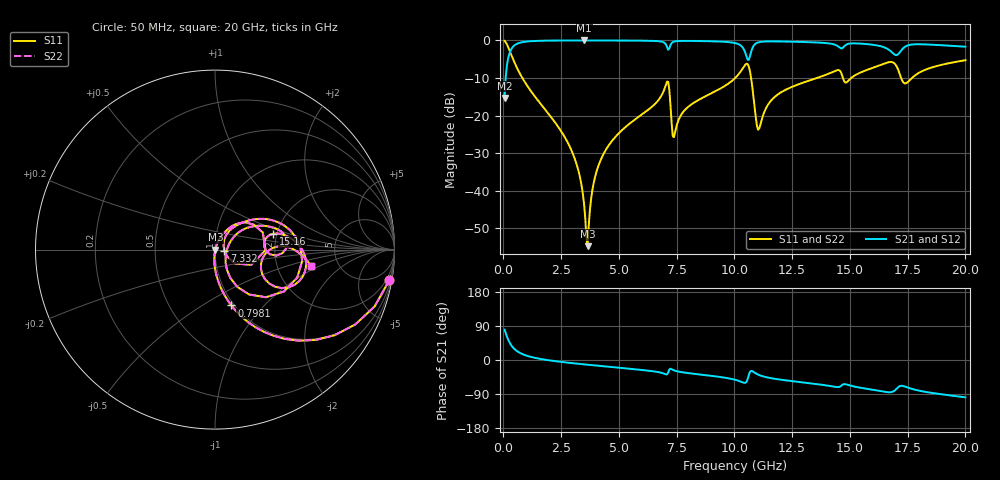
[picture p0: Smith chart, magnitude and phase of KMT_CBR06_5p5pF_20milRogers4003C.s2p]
! Data measured by Modelithics Inc. support@modelithics.com 813-866-6335
! KEMET CBR0603 5.5pF, Pad Width= 0.851mm, Pad Length= 0.64mm, Pad Gap= 0.62mm, 20mil Rogers 4003C substrate Data, January 2022
# hz S ma R 50
! 2 Port Network Data from SP1.SP block
! freq  magS11  angS11  magS21  angS21  magS12  angS12  magS22  angS22
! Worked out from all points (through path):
!   401 points, 50 MHz to 20 GHz, reference 50 ohm
!   highest |S21| = -0.02 dB at 3.491 GHz (marker M1); lowest = -15.3 dB at 50 MHz (marker M2)
!   group delay of S21, straight-line fit = 15.3 ps
!   lowest |S11| = -54.7 dB at 3.641 GHz (marker M3), VSWR 1.00, Z = 50.2 + j0.024 ohm
!   |S11| at or under -10 dB: 818.8 MHz to 10.03 GHz (9.214 GHz wide, 170 % of centre); 10.72 GHz to 13.57 GHz (2.851 GHz wide, 23.5 % of centre); 17.22 GHz to 17.69 GHz (468.5 MHz wide, 2.68 % of centre)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
!   |S22| runs from -54.7 to -0.1 dB; largest |S21 - S12| = 0
!   S11 on the Smith chart (normalised r, x): 50 MHz: 1, -11; 798.1 MHz: 0.97, -0.67; 7.332 GHz: 1.11, -0.01; 15.16 GHz: 1.90, +0.38; 20 GHz: 3.15, -0.84
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5e7  0.9851 -10.1  0.1717 79.9  0.1717 79.9  0.9851 -10.1
2.99375e8  0.6893 -47.4  0.7238 42.6  0.7238 42.6  0.6893 -47.4
7.98125e8  0.3242 -73.7  0.9451 16.2  0.9451 16.2  0.3242 -73.7
2.74325e9  0.04616 -94.9  0.9973 -6.7  0.9973 -6.7  0.04616 -94.9
3.391625e9  0.0113 -92.5  0.9982 -10.9  0.9982 -10.9  0.0113 -92.5
3.491375e9  0.006594 -86.8  0.9982 -11.6  0.9982 -11.6  0.006594 -86.8
3.641e9  0.001833 7.5  0.9981 -12.5  0.9981 -12.5  0.001833 7.5
3.94025e9  0.01415 68.4  0.998 -14.3  0.998 -14.3  0.01415 68.4
4.389125e9  0.03321 69.8  0.9974 -16.9  0.9974 -16.9  0.03321 69.8
6.73325e9  0.1641 53.7  0.9749 -32.3  0.9749 -32.3  0.1641 53.7
7.082375e9  0.2829 19.7  0.8191 -37.9  0.8191 -37.9  0.2829 19.7
7.33175e9  0.05307 -6.6  0.9495 -25.9  0.9495 -25.9  0.05307 -6.6
1.0025e10  0.3145 33.0  0.9224 -52.1  0.9224 -52.1  0.3145 33.0
1.057362e10  0.4839 -18.9  0.5539 -50.1  0.5539 -50.1  0.4839 -18.9
1.0823e10  0.1802 -61.6  0.84 -31.2  0.84 -31.2  0.1802 -61.6
1.107238e10  0.06717 1.5  0.9482 -39.8  0.9482 -39.8  0.06717 1.5
1.177062e10  0.18 35.9  0.9699 -49.8  0.9699 -49.8  0.18 35.9
1.336662e10  0.3013 26.1  0.9438 -62.2  0.9438 -62.2  0.3013 26.1
1.516212e10  0.3345 15.2  0.9133 -69.8  0.9133 -69.8  0.3345 15.2
1.670825e10  0.5142 -9.2  0.7418 -85.2  0.7418 -85.2  0.5142 -9.2
1.74065e10  0.2678 -12.8  0.8303 -70.5  0.8303 -70.5  0.2678 -12.8
2e10  0.5451 -9.9  0.8239 -98.5  0.8239 -98.5  0.5451 -9.9
